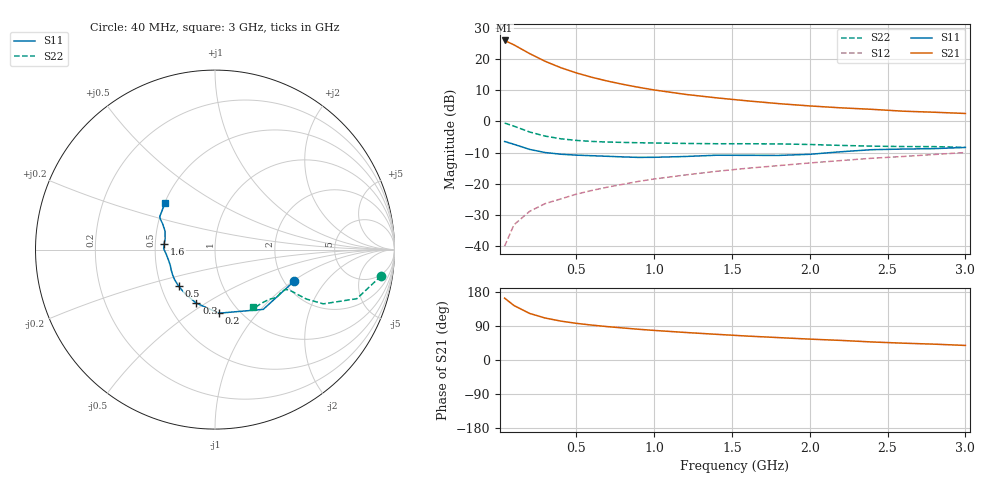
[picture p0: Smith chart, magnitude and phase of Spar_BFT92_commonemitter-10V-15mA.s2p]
! Filename:  BFT92I.S2P  Version:  2.0
! NXP part #: BFT92  Date: May 1990
! Bias condition: Vce=-10V, Ic=-15mA
#  MHz  S  MA  R  50
! Freq  S11  S21  S12  S22  !GUM [dB]
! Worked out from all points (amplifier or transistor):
!   21 points, 40 MHz to 3 GHz, reference 50 ohm
!   highest |S21| = 25.9 dB at 40 MHz (marker M1)
!   |S21| within 3 dB of that: start of sweep to 157.2 MHz
!   unconditionally stable (mu >= 1): 664.9 MHz to 2.327 GHz
!   at 300 MHz: K = 0.77, MSG = 22.8 dB, |S12| = -26.4 dB
!   at 1 GHz: K = 1.06, MAG = 12.8 dB, |S12| = -18.5 dB
!   at 3 GHz: K = 0.94, MSG = 6.3 dB, |S12| = -10.0 dB
!   S11 on the Smith chart (normalised r, x): 40 MHz: 2.26, -1.02; 200 MHz: 0.81, -0.66; 300 MHz: 0.69, -0.46; 500 MHz: 0.62, -0.27; 1.6 GHz: 0.56, +0.04; 3 GHz: 0.50, +0.30
40  0.475 -21.7  19.7 163.2  0.01 81.5  0.937 -9.0
100  0.428 -51.1  16.75 143.8  0.022 72.4  0.836 -19.1
200  0.355 -86.3  12.16 123.0  0.036 67.0  0.675 -26.6
300  0.316 -109.2  9.143 110.8  0.048 66.7  0.579 -28.4
400  0.297 -124.4  7.231 102.7  0.057 67.3  0.525 -28.5
500  0.287 -135.0  5.962 96.8  0.068 68.2  0.494 -28.5
600  0.281 -143.0  5.069 92.1  0.078 69.1  0.476 -28.6
700  0.275 -149.2  4.409 88.1  0.088 69.7  0.465 -28.8
800  0.269 -155.1  3.904 84.5  0.098 70.2  0.459 -29.1
900  0.264 -160.7  3.504 81.1  0.109 70.3  0.453 -29.4
1000  0.265 -165.8  3.177 78.1  0.119 70.4  0.449 -30.1
1200  0.273 -174.7  2.7 72.7  0.138 70.3  0.442 -31.6
1400  0.286 179.0  2.375 67.8  0.158 70.2  0.437 -33.6
1600  0.285 174.0  2.123 63.1  0.177 69.7  0.437 -35.5
1800  0.284 168.0  1.918 59.1  0.195 69.4  0.434 -37.6
2000  0.296 159.9  1.762 55.1  0.215 68.8  0.425 -39.6
2200  0.325 153.8  1.642 51.7  0.235 68.2  0.411 -42.3
2400  0.351 150.6  1.554 47.6  0.256 67.4  0.4 -46.5
2600  0.359 148.9  1.451 44.4  0.273 66.7  0.394 -50.8
2800  0.365 144.1  1.396 41.8  0.294 66.5  0.393 -53.9
3000  0.381 137.2  1.334 38.4  0.316 65.6  0.382 -56.7
